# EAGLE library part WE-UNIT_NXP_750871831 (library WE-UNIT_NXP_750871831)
Off-Line Transformer WE-Unit NXP - Nominal input voltage: 85-265 VAC - Operating temperature: -40°C to +125 °C - Isolation voltage 4 kVAC -- Especially designed for several ICs from NXP TEA1623PH -- Universal input -- Smart meters -- Dimmable 12 V LED driver -- Offline-switch mode power supplies
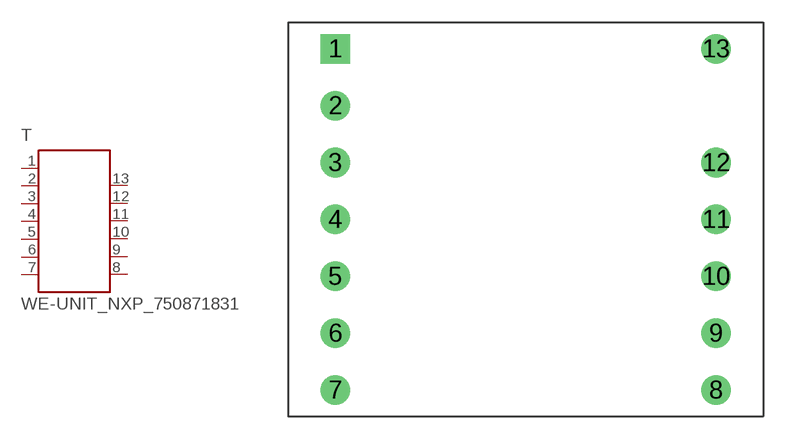
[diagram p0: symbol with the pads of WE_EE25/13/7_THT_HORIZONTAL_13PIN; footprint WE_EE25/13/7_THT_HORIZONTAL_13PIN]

Designator prefix T

## WE-UNIT_NXP_750871831 (MPN: 750871831; OC_FARNELL: 1849058; OC_NEWARK: 13T9848; PACKAGE: EE25_13_7; SUPPLIER: Würth Elektronik eiSos GmbH)  [WE_EE25/13/7_THT_HORIZONTAL_13PIN]
1  1  pas
2  2  pas
3  3  pas
4  4  pas
5  5  pas
6  6  pas
7  7  pas
8  8  pas
9  9  pas
10  10  pas
11  11  pas
12  12  pas
13  13  pas

## Footprint WE_EE25/13/7_THT_HORIZONTAL_13PIN (pad centres in mm)
Transformer, EE25/13/7 THT Horizontal 13 Pin
drill 1.32 square: 1 -12.75,11.43
drill 1.32: 2 -12.75,7.62; 3 -12.75,3.81; 4 -12.75,0; 5 -12.75,-3.81; 6 -12.75,-7.62; 7 -12.75,-11.43; 8 12.75,-11.43; 9 12.75,-7.62; 10 12.75,-3.81; 11 12.75,0; 12 12.75,3.81; 13 12.75,11.43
